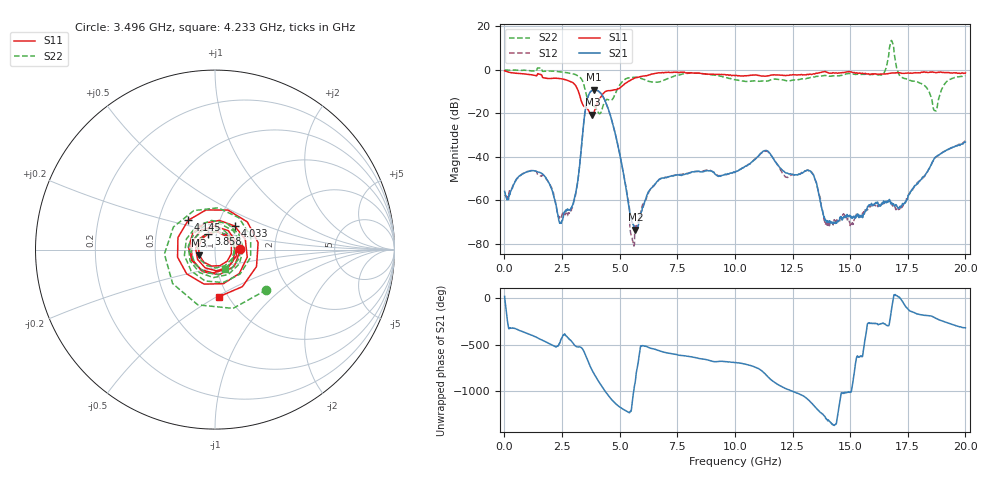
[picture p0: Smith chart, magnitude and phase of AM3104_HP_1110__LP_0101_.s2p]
!Created with skrf (http://scikit-rf.org).
# Hz S RI R 50.0
!freq ReS11 ImS11 ReS21 ImS21 ReS12 ImS12 ReS22 ImS22
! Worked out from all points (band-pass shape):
!   1601 points, 10 MHz to 20 GHz, reference 50 ohm
!   highest |S21| = -9.15 dB at 3.896 GHz (marker M1); lowest = -73.4 dB at 5.682 GHz (marker M2)
!   |S21| within 3 dB of the highest: 3.633 GHz to 4.272 GHz (639.5 MHz wide, 16.2 % of centre)
!   lowest |S11| = -20.6 dB at 3.821 GHz (marker M3), VSWR 1.21, Z = 41.9 - j2.68 ohm
!   |S11| at or under -10 dB: 3.216 GHz to 4.371 GHz (1.155 GHz wide, 30.4 % of centre)
!   |S22| runs from -20.1 to 13.5 dB; largest |S21 - S12| = 0.021
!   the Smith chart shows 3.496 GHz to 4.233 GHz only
!   S11 on the Smith chart (normalised r, x): 3.496 GHz: 1.33, +0.00; 3.858 GHz: 0.91, +0.17; 4.033 GHz: 1.20, +0.32; 4.145 GHz: 0.71, +0.24; 4.233 GHz: 0.91, -0.51
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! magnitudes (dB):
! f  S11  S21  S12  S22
! 10 MHz  -0.4  -55.8  -57.9  -0.1
! 1.572 GHz  -2.1  -47.3  -48.7  0.8
! 2.459 GHz  -4.1  -70.5  -67.7  -0.9
! 2.984 GHz  -6.0  -61.3  -62.1  -1.8
! 3.346 GHz  -14.6  -35.0  -35.0  -4.2
! 3.496 GHz  -17.0  -19.5  -19.5  -8.8
! 3.821 GHz  -20.6  -9.4  -9.4  -16.3
! 3.858 GHz  -20.3  -9.2  -9.2  -16.7
! 3.896 GHz  -19.2  -9.2  -9.2  -16.7
! 4.033 GHz  -15.3  -9.5  -9.5  -18.9
! 4.145 GHz  -13.1  -10.3  -10.4  -20.1
! 4.233 GHz  -11.6  -11.5  -11.5  -18.3
! 5.545 GHz  -4.3  -70.2  -77.6  -3.5
! 5.682 GHz  -3.7  -73.4  -71.7  -3.4
! 6.682 GHz  -1.4  -50.8  -50.7  -5.6
! 10.01 GHz  -2.7  -47.1  -46.9  -4.5
! 11.33 GHz  -2.9  -37.1  -37.4  -5.1
! 13.34 GHz  -2.1  -47.4  -47.1  -3.5
! 14.02 GHz  -1.2  -70.0  -70.9  -2.7
! 16.68 GHz  -1.6  -60.3  -60.6  7.1
! 18.69 GHz  -1.2  -40.2  -40.3  -18.8
! 20 GHz  -1.4  -33.2  -32.7  -2.6
